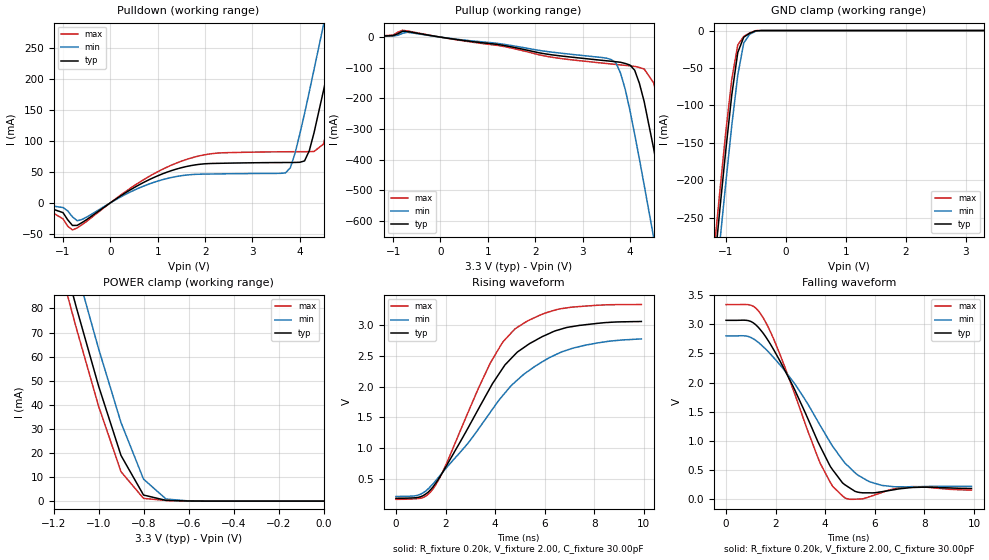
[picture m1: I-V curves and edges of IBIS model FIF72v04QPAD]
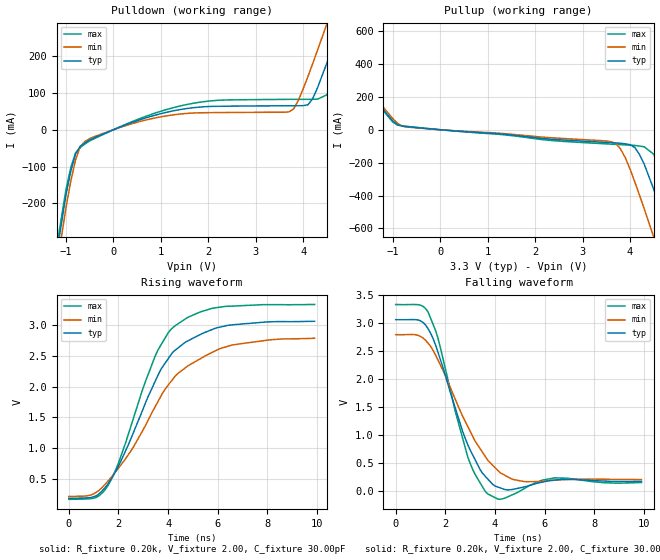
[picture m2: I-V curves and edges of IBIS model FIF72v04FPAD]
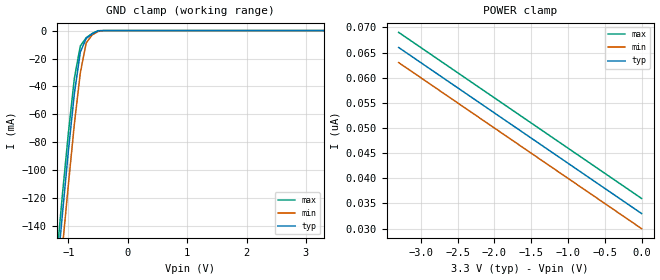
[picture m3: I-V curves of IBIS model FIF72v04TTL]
| IBIS file i72v83.ibs created by s2ibis2 version 1.1
| North Carolina State University Electronics Research Laboratory  1995
[IBIS ver]   2.1
[File name]   i72v83.ibs
[File Rev]   1.0
[Date]   07/15/98
[Source]   Integrated Device Technology, Inc.
[Notes]   1. Temperatures: typ=25C, min=70C, max=0C 2. Cemos8_5v
   process. 3. Ramp rates based on 50 ohm load.
[Copyright]   Copyright 1997, Integrated Device Technology, Inc.
|   Component idt72V83
[Component]   idt72V83
[Manufacturer]   Integrated Device Technology
[Package]
| variable   typ   min   max
R_pkg   0.75   0.60   0.90
L_pkg   8.10nH   8.30nH   9.90nH
C_pkg   0.53pF   0.46pF   0.60pF
[Pin]  signal_name   model_name   R_pin   L_pin   C_pin
1   FFAL   FIF72v04FPAD
2   QA0   FIF72v04QPAD
3   QA1   FIF72v04QPAD
4   QA2   FIF72v04QPAD
5   QA3   FIF72v04QPAD
6   QA8   FIF72v04QPAD
7   GND   GND
8   RAL   FIF72v04TTL
9   QA4   FIF72v04QPAD
10   QA5   FIF72v04QPAD
11   QA6   FIF72v04QPAD
12   QA7   FIF72v04QPAD
13   XOLHFAL   FIF72v04FPAD
14   EFAL   FIF72v04FPAD
15   FFBL   FIF72v04FPAD
16   QB0   FIF72v04QPAD
17   QB1   FIF72v04QPAD
18   QB2   FIF72v04QPAD
19   QB3   FIF72v04QPAD
20   QB8   FIF72v04QPAD
21   GND   GND
22   RBL   FIF72v04TTL
23   QB4   FIF72v04QPAD
24   QB5   FIF72v04QPAD
25   QB6   FIF72v04QPAD
26   QB7   FIF72v04QPAD
27   XOLHFBL   FIF72v04FPAD
28   EFBL   FIF72v04FPAD
29   RSBL   FIF72v04TTL
30   FLRTBL   FIF72v04TTL
31   DB7   FIF72v04TTL
32   DB6   FIF72v04TTL
33   DB5   FIF72v04TTL
34   DB4   FIF72v04TTL
35   VCC   POWER
36   WBL   FIF72v04TTL
37   DB8   FIF72v04TTL
38   DB3   FIF72v04TTL
39   DB2   FIF72v04TTL
40   DB1   FIF72v04TTL
41   DB0   FIF72v04TTL
42   XIBL   FIF72v04TTL
43   RSAL   FIF72v04TTL
44   FLRTAL   FIF72v04TTL
45   DA7   FIF72v04TTL
46   DA6   FIF72v04TTL
47   DA5   FIF72v04TTL
48   DA4   FIF72v04TTL
49   VCC   POWER
50   WAL   FIF72v04TTL
51   DA8   FIF72v04TTL
52   DA3   FIF72v04TTL
53   DA2   FIF72v04TTL
54   DA1   FIF72v04TTL
55   DA0   FIF72v04TTL
56   XIAL   FIF72v04TTL
| Models and submodels in the file (3): FIF72v04QPAD (3-state), FIF72v04FPAD (Output), FIF72v04TTL (Input)
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| FIN  FIN   dummy_model
| QIN  QIN   dummy_model
| QOEL QOEL   dummy_model
|   Model FIF72v04QPAD
[Model]   FIF72v04QPAD
Model_type   3-state
Polarity   Non-Inverting
Enable   Active-Low
Vmeas =  1.500V
C_comp   3.00pF   NA   NA
[Temperature Range]   25.00   70.00   0.000
[Voltage Range]   3.30V   3.00V   3.60V
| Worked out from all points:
|   slope of the pulldown table from 0 to 0.495 V, typ, clamps not added: 20.4 ohm
|   slope of the pullup table from 0 to 0.495 V, typ, clamps not added: 44.7 ohm
|   GND clamp passes 1 mA (typ) near -0.52 V on its own axis
|   POWER clamp passes 1 mA (typ) near -0.73 V on its own axis
|   rising waveform, R_fixture 0.20k, V_fixture 2.00, C_fixture 30.00pF: 20-80 % time 2.61ns typ, 3.24ns min, 2.18ns max; typ from 0.181 V to 3.06 V
|   falling waveform, R_fixture 0.20k, V_fixture 2.00, C_fixture 30.00pF: 20-80 % time 1.95ns typ, 2.38ns min, 1.67ns max; typ from 3.07 V to 0.18 V
[Pulldown]
| voltage   I(typ)   I(min)   I(max)
-3.3V     -1mA       -1mA       0A
-1.5V     -2.7mA     -2.1mA     -3.3mA
-800mV    -36.55mA   -22.69mA   -43.77mA
1.5V      56.64mA    43.75mA    67.16mA
3.7V      65mA       48.37mA    82.35mA
3.9V      65.11mA    80.12mA    82.43mA
4.1V      67.6mA     144mA      82.48mA
4.5V      181mA      287mA      94.75mA
4.7V      253mA      361mA      155mA
4.9V      326mA      435mA      225mA
5.1V      400mA      510mA      298mA
6.6V      966mA      1.076A     862mA
[Pullup]
| voltage   I(typ)   I(min)   I(max)
-3.3V     300uA      300uA      300uA
-800mV    19.13mA    12.44mA    22.38mA
3.6V      -78.68mA   -72.88mA   -87.52mA
3.7V      -80.24mA   -82.94mA   -89.09mA
3.9V      -85.87mA   -170mA     -92.22mA
4.1V      -108mA     -317mA     -95.4mA
4.3V      -210mA     -482mA     -104mA
4.5V      -363mA     -653mA     -149mA
4.7V      -531mA     -826mA     -270mA
4.9V      -703mA     -1A        -430mA
5.1V      -878mA     -1.176A    -601mA
6.6V      -2.207A    -2.508A    -1.926A
[GND_clamp]
| voltage   I(typ)   I(min)   I(max)
-3.3V     -2.171A    -2.212A    -2.149A
-1.2V     -323mA     -367mA     -298mA
-1.1V     -240mA     -284mA     -216mA
-1V       -160mA     -204mA     -136mA
-900mV    -86.07mA   -127mA     -65.05mA
-800mV    -29.34mA   -59.59mA   -19.24mA
-700mV    -8.788mA   -16.49mA   -7.804mA
-600mV    -3.672mA   -4.887mA   -3.17mA
-500mV    -365uA     -944uA     -138uA
-400mV    -14.29nA   -611nA     -4.611nA
3.3V      33nA       33.88nA    33nA
[POWER_clamp]
| voltage   I(typ)   I(min)   I(max)
-3.3V     901mA      915mA      893mA
-1.2V     116mA      132mA      107mA
-1.1V     80.92mA    96.84mA    72.29mA
-1V       47.89mA    63.39mA    39.51mA
-900mV    18.95mA    32.6mA     12.21mA
-800mV    2.533mA    9.147mA    1.14mA
-700mV    314uA      878uA      268uA
-600mV    64.82uA    96.03uA    58.5uA
0V        33nA       30nA       36nA
[Ramp]
| variable   typ   min   max
dV/dt_r   1.03/1.78n   0.87/2.19n   1.19/1.55n
dV/dt_f   1.35/1.74n   1.12/2.29n   1.54/1.44n
R_load = 50.00
[Rising Waveform]
R_fixture = 0.20k
V_fixture = 2.00
C_fixture = 30.00pF
R_dut = 0.75
L_dut = 8.10nH
C_dut = 0.53pF
| time   V(typ)   V(min)   V(max)
0s        181mV      211mV      165mV
900ps     197mV      234mV      177mV
1.5ns     369mV      418mV      337mV
1.9ns     615mV      612mV      624mV
3.8ns     1.978V     1.577V     2.377V
4.3ns     2.292V     1.848V     2.717V
4.8ns     2.52V      2.07V      2.937V
6.7ns     2.938V     2.565V     3.268V
8.1ns     3.026V     2.707V     3.321V
9.9ns     3.058V     2.774V     3.334V
[Falling Waveform]
R_fixture = 0.20k
V_fixture = 2.00
C_fixture = 30.00pF
R_dut = 0.75
L_dut = 8.10nH
C_dut = 0.53pF
| time   V(typ)   V(min)   V(max)
0s        3.068V     2.8V       3.338V
1ns       3.048V     2.773V     3.327V
1.5ns     2.845V     2.613V     3.108V
2.8ns     1.847V     1.961V     1.769V
3.8ns     901mV      1.261V     611mV
4.3ns     501mV      905mV      217mV
4.8ns     243mV      615mV      17.16mV
6.3ns     126mV      233mV      114mV
7.5ns     197mV      210mV      213mV
9.9ns     180mV      216mV      154mV
|   Model FIF72v04FPAD
[Model]   FIF72v04FPAD
Model_type   Output
Vmeas =  1.500V
C_comp   3.00pF   NA   NA
[Temperature Range]   25.00   70.00   0.000
[Voltage Range]   3.30V   3.00V   3.60V
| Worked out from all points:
|   slope of the pulldown table from 0 to 0.495 V, typ, clamps not added: 20.4 ohm
|   slope of the pullup table from 0 to 0.495 V, typ, clamps not added: 44.7 ohm
|   rising waveform, R_fixture 0.20k, V_fixture 2.00, C_fixture 30.00pF: 20-80 % time 2ns typ, 2.49ns min, 1.71ns max; typ from 0.181 V to 3.07 V
|   falling waveform, R_fixture 0.20k, V_fixture 2.00, C_fixture 30.00pF: 20-80 % time 1.28ns typ, 1.68ns min, 1.07ns max; typ from 3.07 V to 0.177 V
[Pulldown]
| voltage   I(typ)   I(min)   I(max)
-3.3V     -2.791A    -2.213A    -2.149A
-1.5V     -582mA     -626mA     -558mA
-1V       -176mA     -211mA     -162mA
-800mV    -65.89mA   -82.28mA   -63.01mA
-400mV    -21.63mA   -18.48mA   -23.86mA
1.6V      58.46mA    44.74mA    69.8mA
3.7V      65mA       48.37mA    82.35mA
4.1V      67.6mA     144mA      82.48mA
4.5V      181mA      287mA      94.75mA
4.7V      253mA      361mA      155mA
5.1V      400mA      510mA      298mA
6.6V      966mA      1.076A     862mA
[Pullup]
| voltage   I(typ)   I(min)   I(max)
-3.3V     901mA      915mA      893mA
-2.5V     598mA      613mA      590mA
-900mV    29.8mA     38.77mA    28.31mA
3.6V      -78.68mA   -72.88mA   -87.52mA
3.9V      -85.87mA   -170mA     -92.22mA
4.1V      -108mA     -317mA     -95.4mA
4.3V      -210mA     -482mA     -104mA
4.5V      -363mA     -653mA     -149mA
4.7V      -531mA     -826mA     -270mA
4.9V      -703mA     -1A        -430mA
5.1V      -878mA     -1.176A    -601mA
6.6V      -2.207A    -2.508A    -1.926A
[Ramp]
| variable   typ   min   max
dV/dt_r   1.03/1.15n   0.87/1.36n   1.19/1.05n
dV/dt_f   1.35/0.80n   1.13/1.03n   1.54/0.68n
R_load = 50.00
[Rising Waveform]
R_fixture = 0.20k
V_fixture = 2.00
C_fixture = 30.00pF
R_dut = 0.75
L_dut = 8.10nH
C_dut = 0.53pF
| time   V(typ)   V(min)   V(max)
0s        181mV      211mV      165mV
1.1ns     221mV      278mV      196mV
1.6ns     430mV      472mV      405mV
2ns       708mV      674mV      758mV
2.6ns     1.25V      1.015V     1.482V
3.5ns     2.107V     1.69V      2.521V
4.3ns     2.599V     2.181V     2.998V
5.3ns     2.851V     2.455V     3.218V
6.6ns     3.008V     2.681V     3.313V
9.9ns     3.066V     2.79V      3.339V
[Falling Waveform]
R_fixture = 0.20k
V_fixture = 2.00
C_fixture = 30.00pF
R_dut = 0.75
L_dut = 8.10nH
C_dut = 0.53pF
| time   V(typ)   V(min)   V(max)
0s        3.068V     2.8V       3.338V
900ps     3.063V     2.788V     3.336V
1.3ns     2.91V      2.65V      3.208V
1.7ns     2.489V     2.349V     2.742V
2.9ns     837mV      1.163V     619mV
3.7ns     223mV      559mV      -45.13mV
4.2ns     62.68mV    334mV      -144mV
5.2ns     79.41mV    172mV      53.13mV
6.4ns     200mV      197mV      239mV
9.9ns     177mV      210mV      157mV
|   Model FIF72v04TTL
[Model]   FIF72v04TTL
Model_type   Input
Vinl =  0.000V
Vinh =  3.000V
Vmeas =  1.500V
C_comp   3.00pF   NA   NA
[Temperature Range]   25.00   70.00   0.000
[Voltage Range]   3.30V   3.00V   3.60V
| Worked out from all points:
|   GND clamp passes 1 mA (typ) near -0.54 V on its own axis
[GND_clamp]
| voltage   I(typ)   I(min)   I(max)
-3.3V     -1.215A    -1.238A    -1.203A
-1.2V     -177mA     -201mA     -164mA
-1.1V     -131mA     -155mA     -117mA
-1V       -85.93mA   -110mA     -73.12mA
-900mV    -45.18mA   -67.04mA   -34.18mA
-800mV    -15.46mA   -30.4mA    -11.09mA
-700mV    -5.585mA   -8.799mA   -5.095mA
-600mV    -2.402mA   -3.119mA   -2.049mA
-500mV    -211uA     -600uA     -61.98uA
-400mV    -8.305nA   -258nA     -4.256nA
3.3V      33nA       33nA       33nA
[POWER_clamp]
| voltage   I(typ)   I(min)   I(max)
-3.3V     66nA       63nA       69nA
-3.2V     65nA       62nA       68nA
-3V       63nA       60nA       66nA
0V        33nA       30nA       36nA
